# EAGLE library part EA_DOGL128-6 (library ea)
ELECTRONIC ASSEMBLY GmbH EA DOGL128B-6 EA DOGL128E-6 EA DOGL128L-6 EA DOGL128W-6 EA DOGL128S-6
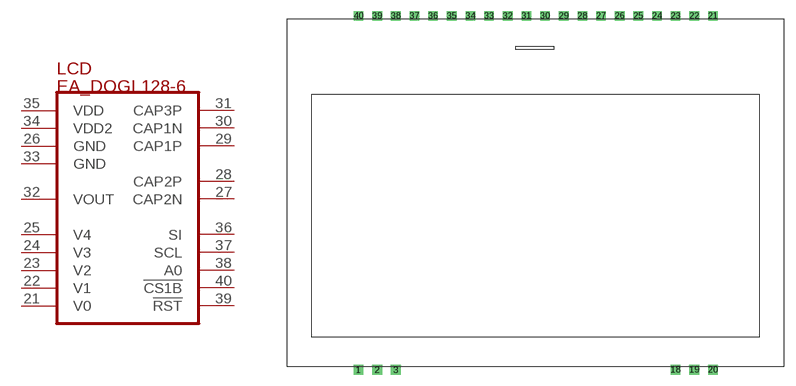
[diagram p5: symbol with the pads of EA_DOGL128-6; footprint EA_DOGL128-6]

Designator prefix LCD

## EA_DOGL128-6  [EA_DOGL128-6]
21  V0  in
22  V1  in
23  V2  pas
24  V3  pas
25  V4  pas
26  GND
27  CAP2N
28  CAP2P
29  CAP1P
30  CAP1N
31  CAP3P
32  VOUT  pas
33  GND
34  VDD2  pwr
35  VDD  pwr
36  SI
37  SCL  in
38  A0  in
39  !RST!  in
40  !CS1B!  in

## Footprint EA_DOGL128-6 (pad centres in mm)
EA DOGL128-6 Grafikdisplay COG 128x64 Pixel inkl.Kontroller Hersteller: ELECTRONIC ASSEMBLY GmbH http://www.lcd-module.de
drill 0.813 square: 1 0,0; 2 2.54,0; 3 5.08,0; 18 43.18,0; 19 45.72,0; 20 48.26,0; 21 48.26,48.26; 22 45.72,48.26; 23 43.18,48.26; 24 40.64,48.26; 25 38.1,48.26; 26 35.56,48.26; 27 33.02,48.26; 28 30.48,48.26; 29 27.94,48.26; 30 25.4,48.26; 31 22.86,48.26; 32 20.32,48.26; 33 17.78,48.26; 34 15.24,48.26; 35 12.7,48.26; 36 10.16,48.26; 37 7.62,48.26; 38 5.08,48.26; 39 2.54,48.26; 40 0,48.26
